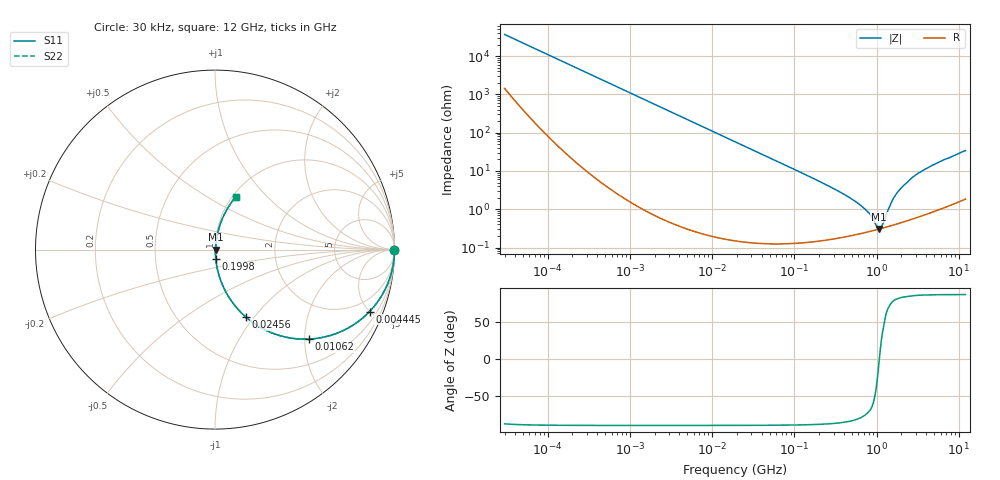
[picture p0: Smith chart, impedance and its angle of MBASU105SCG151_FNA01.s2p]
! MBASU105SCG151_FNA01  S-PARAMETER MODEL  ( General Type )
! Model Generated by TAIYO YUDEN Corporation (http://www.ty-top.com)
! Version 1.0
! TAIYO YUDEN Control No. 130207
! Copyright(c) 2013 TAIYO YUDEN CO.,LTD. All Rights Reserved.
! Product Description (link to TY-COMPAS)
! https://ds.yuden.co.jp/TYCOMPAS/or/detail?pn=MBASU105SCG151JFNA01&u=M
! Products Name : Multilayer Ceramic Capacitors
! Characteristics :
!  Capacitance : 150 pF , Rated Voltage : 50V , TCC : CG / C0G
!  Case Size : 1.0 x 0.5 / 0.039 x 0.02 [mm/inch] , Thickness : 0.5 / 0.02 [mm/inch]
!  (Conditions: Temperature = 25 degC , DC Bias Current/Voltage = 0A / 0V)
! External Node Assignments :
!  1  o---| |---o  2
! GND o---------o GND
! Frequency Range : 30000Hz  -  12GHz  [ 401 STEP ]
# MHz S RI R 50
! Freq[MHz].  S11 Real  S11 Imag  S21 Real  S21 Imag  S12 Real  S12 Imag  S22 Real  S22 Imag
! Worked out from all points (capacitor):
!   401 points, 30 kHz to 12 GHz, reference 50 ohm
!   read as one part in series: C = 144 pF near 32 kHz
!   lowest |Z| = 304 mohm at 1.069 GHz (marker M1)
!   series resonance near 1.079 GHz, so ESL is about 150 pH
!   S11 on the Smith chart (normalised r, x): 30 kHz: open; 4.445 MHz: 1.01, -4.99; 10.62 MHz: 1.00, -2.09; 24.56 MHz: 1.00, -0.90; 199.8 MHz: 1.00, -0.11; 12 GHz: 1.04, +0.68
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0.03  0.9999 -0.0027  0.000112 0.0027  0.000112 0.0027  0.9999 -0.0027
0.260295  0.9994 -0.0235  0.000619 0.0235  0.000619 0.0235  0.9994 -0.0235
0.886466  0.9935 -0.0794  0.00647 0.0794  0.00647 0.0794  0.9935 -0.0794
2.258455  0.9599 -0.1955  0.0401 0.1955  0.0401 0.1955  0.9599 -0.1955
4.445489  0.8612 -0.3451  0.1388 0.3451  0.1388 0.3451  0.8612 -0.3451
10.61839  0.5215 -0.4986  0.4785 0.4986  0.4785 0.4986  0.5215 -0.4986
18.97367  0.255 -0.4346  0.745 0.4346  0.745 0.4346  0.255 -0.4346
24.55797  0.1699 -0.3741  0.8301 0.3741  0.8301 0.3741  0.1699 -0.3741
51.55976  0.0451 -0.2047  0.9549 0.2047  0.9549 0.2047  0.0451 -0.2047
164.6252  0.00573 -0.0656  0.9943 0.0656  0.9943 0.0656  0.00573 -0.0656
199.7686  0.00436 -0.0536  0.9956 0.0536  0.9956 0.0536  0.00436 -0.0536
617.6002  0.00244 -0.0131  0.9976 0.0131  0.9976 0.0131  0.00244 -0.0131
825.5698  0.00267 -0.00705  0.9973 0.00705  0.9973 0.00705  0.00267 -0.00705
1001.808  0.00292 -0.00198  0.9971 0.00198  0.9971 0.00198  0.00292 -0.00198
1068.55  0.00302 -0.000272  0.997 0.000272  0.997 0.000272  0.00302 -0.000272
1177.092  0.0032 0.00227  0.9968 -0.00227  0.9968 -0.00227  0.0032 0.00227
1428.372  0.0037 0.0107  0.9963 -0.0107  0.9963 -0.0107  0.0037 0.0107
1625.032  0.00429 0.0199  0.9957 -0.0199  0.9957 -0.0199  0.00429 0.0199
1848.769  0.0051 0.0295  0.9949 -0.0295  0.9949 -0.0295  0.0051 0.0295
2903.719  0.0112 0.0734  0.9888 -0.0734  0.9888 -0.0734  0.0112 0.0734
5715.613  0.0371 0.1628  0.9629 -0.1628  0.9629 -0.1628  0.0371 0.1628
12000  0.1166 0.2951  0.8834 -0.2951  0.8834 -0.2951  0.1166 0.2951
